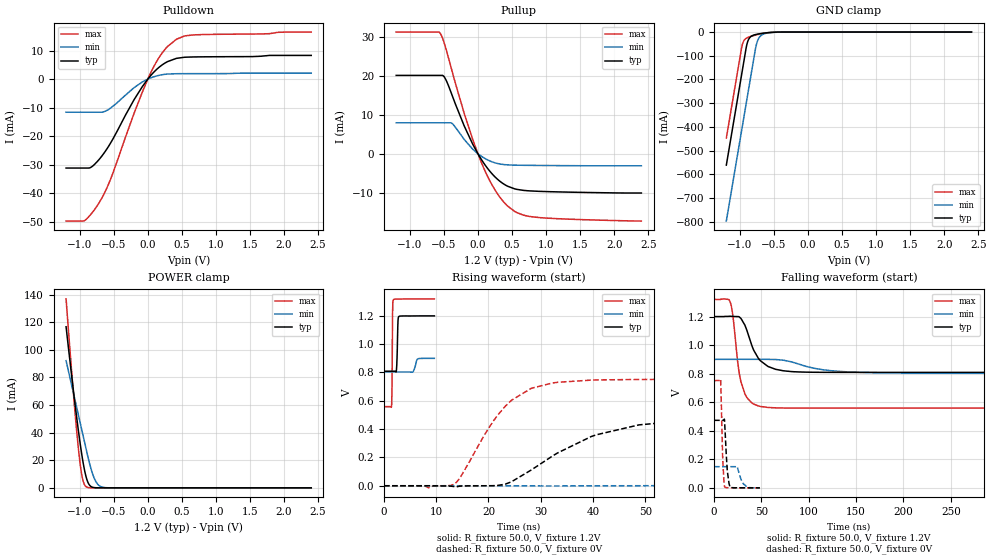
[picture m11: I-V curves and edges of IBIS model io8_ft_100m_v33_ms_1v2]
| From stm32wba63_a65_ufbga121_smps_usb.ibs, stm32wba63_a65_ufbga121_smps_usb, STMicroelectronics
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[Model]   io8_ft_100m_v33_ms_1v2
Model_type I/O
Polarity   Non-Inverting
Enable   Active-Low
| CAP_THRESHOLD on pad IOFT is "UDTCAPC" :
| Rising=30.0% of vddiom   Falling=70.0% of vddiom
| C_comp min and max val. don't necessarily correlate with the min and max pvt
| but are the smallest and greatest pad capacitance found.
| var   typ   min   max
C_comp   2.93788pF  2.85554pF  3.04885pF
|C_comp_pullup   1.70472pF  1.54555pF  1.84622pF
|C_comp_pulldown   1.23316pF  1.30998pF  1.20263pF
Vinl = 450.0mV
Vinh = 660.0mV
Vmeas = 600.0mV   | Reference voltage for timing measurements
Cref  = 50.0pF   | Timing specification test load capacitance value
Rref  = 1.0MOhm   | Timing specification test load resistance value
Vref  = 660.0mV   | Timing specification test load voltage
[Model Spec]
| TIME_THRESHOLD on pin ZIV33M is "CMOS" :
| Rising=50.0% of vddiom   Falling=50.0% of vddiom
Vinl 436.50000mV 331.50000mV 482.50000mV
Vinh 753.50000mV 549.50000mV 837.50000mV
| variable   typ   min   max
[Temperature Range] 25.0 140.0 -40.0
| variable   typ   min   max
[Voltage Range] 1.2V 900.0mV 1.32V
| variable   typ   min   max
[POWER Clamp Reference] 1.2V 900.0mV 1.32V
| variable   typ   min   max
[GND Clamp Reference] 0V 0V 0V
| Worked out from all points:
|   slope of the pulldown table from 0 to 0.18 V, typ, clamps not added: 40.6 ohm
|   slope of the pullup table from 0 to 0.18 V, typ, clamps not added: 39.4 ohm
|   GND clamp passes 1 mA (typ) near -0.51 V on its own axis
|   POWER clamp passes 1 mA (typ) near -0.83 V on its own axis
|   rising waveform, R_fixture 50.0, V_fixture 1.2V: 20-80 % time 157ps typ, 430ps min, 91ps max; typ from 0.809 V to 1.2 V
|   falling waveform, R_fixture 50.0, V_fixture 1.2V: 20-80 % time 16ns typ, 38ns min, 9.4ns max; typ from 1.2 V to 0.809 V
|   rising waveform, R_fixture 50.0, V_fixture 0V: 20-80 % time 15.4ns typ, 36.4ns min, 8.28ns max; typ from 0 V to 0.473 V
|   falling waveform, R_fixture 50.0, V_fixture 0V: 20-80 % time 2.69ns typ, 5.04ns min, 1.95ns max; typ from 0.473 V to 0 V
[POWER Clamp]
-1.2V     116.7mA    92.13mA    136.9mA
-1.09V    69.42mA    68.21mA    67.14mA
-1.02V    41.75mA    52.99mA    28.91mA
-990mV    30.98mA    46.47mA    16.09mA
-970mV    24.36mA    42.12mA    9.575mA
-940mV    15.59mA    35.6mA     3.485mA
-910mV    8.693mA    29.07mA    1.01mA
-860mV    2.259mA    18.59mA    104.6uA
-780mV    143.1uA    6.246mA    2.555uA
-720mV    16.22uA    1.846mA    157.1nA
-650mV    1.267uA    330.3uA    6.118nA
2.4V      0A         0A         0A
[GND Clamp]
-1.2V     -561.6mA   -797.4mA   -447.4mA
-980mV    -187.6mA   -423.4mA   -73.43mA
-960mV    -153.6mA   -389.4mA   -48.26mA
-900mV    -54.17mA   -287.4mA   -24.97mA
-870mV    -29.55mA   -236.4mA   -21.19mA
-830mV    -17.05mA   -168.4mA   -17.42mA
-760mV    -9.921mA   -54.55mA   -11.89mA
-730mV    -8.191mA   -29.78mA   -9.811mA
-690mV    -6.26mA    -14.49mA   -7.318mA
-600mV    -2.976mA   -4.315mA   -3.058mA
-380mV    -57.63uA   -251uA     -19.49uA
2.4V      872.7pA    204.8nA    349.4pA
| variable   typ   min   max
[Pullup Reference] 1.2V 900.0mV 1.32V
| variable   typ   min   max
[Pulldown Reference] 0V 0V 0V
[Pullup]
-1.2V     20.06mA    7.937mA    31.16mA
-580mV    20.06mA    7.937mA    31.16mA
-550mV    20.06mA    7.937mA    30.73mA
-480mV    19.26mA    7.937mA    27.49mA
-380mV    15.01mA    7.757mA    21.16mA
-200mV    7.069mA    3.64mA     10.26mA
20mV      -590.5uA   -260.8uA   -901.4uA
230mV     -5.55mA    -2.199mA   -8.66mA
440mV     -8.335mA   -2.843mA   -13.44mA
570mV     -9.105mA   -2.921mA   -15.05mA
790mV     -9.528mA   -2.972mA   -16.12mA
2.4V      -10.04mA   -3.075mA   -17.21mA
[Pulldown]
-1.2V     -31.2mA    -11.62mA   -49.78mA
-930mV    -31.2mA    -11.62mA   -49.64mA
-830mV    -30.86mA   -11.62mA   -47.25mA
-710mV    -28.04mA   -11.62mA   -43.19mA
-550mV    -22.55mA   -10.2mA    -35.3mA
-200mV    -7.146mA   -2.964mA   -11.89mA
40mV      1.171mA    405.8uA    2.092mA
130mV     3.416mA    1.118mA    6.182mA
230mV     5.302mA    1.613mA    9.763mA
420mV     7.288mA    1.898mA    13.99mA
670mV     7.779mA    1.924mA    15.51mA
2.4V      8.319mA    2.103mA    16.52mA
[Ramp]
dV/dt_r 283.79316mV/14.69967ns 88.92959mV/36.11555ns 450.99229mV/8.2606ns
dV/dt_f 234.65981mV/15.76017ns 57.89579mV/37.90378ns 456.73588mV/9.06629ns
R_load = 50.0
| Removed startup time: 0s 0s 0s  .
| Removed end time: 9.65ns.
[Rising Waveform]
R_fixture   = 50.0
V_fixture   = 1.2V
V_fixture_min = 900.0mV
V_fixture_max = 1.32V
0s        808.9mV    803.5mV    558.8mV
1.45ns    808.9mV    803.5mV    557mV
1.55ns    808.9mV    803.5mV    716.3mV
1.65ns    808.9mV    803.5mV    1.222V
1.8ns     808.9mV    803.5mV    1.313V
2.4ns     820.8mV    803.5mV    1.318V
2.5ns     896.9mV    803.5mV    1.319V
2.65ns    1.127V     803.5mV    1.319V
2.8ns     1.193V     803.5mV    1.318V
9.65ns    1.2V       899.8mV    1.32V
| Removed startup time: 0s 0s 0s  .
| Removed end time: 398.4ns.
[Falling Waveform]
R_fixture   = 50.0
V_fixture   = 1.2V
V_fixture_min = 900.0mV
V_fixture_max = 1.32V
0s        1.2V       900mV      1.32V
17.05ns   1.202V     900mV      1.301V
19.6ns    1.201V     900mV      1.218V
25.3ns    1.2V       900.6mV    863.7mV
28.4ns    1.187V     900.6mV    741.7mV
34.65ns   1.103V     900.5mV    632.4mV
46.8ns    907.1mV    900.2mV    573.8mV
84.95ns   813.2mV    876.4mV    558.9mV
146.4ns   808.9mV    811.1mV    558.8mV
398.4ns   808.9mV    803.5mV    558.8mV
| Removed startup time: 0s 0s 0s  .
| Removed end time: 398.35ns.
[Rising Waveform]
R_fixture   = 50.0
V_fixture   = 0V
V_fixture_min = 0V
V_fixture_max = 0V
0s        4.831nV    215.5nV    3.391nV
13.25ns   -4.891mV   183nV      8.354mV
20.8ns    235uV      21.56nV    449.3mV
24.4ns    27.96mV    22.17uV    603.6mV
28.2ns    111.6mV    -705.9uV   688.3mV
39.65ns   347.3mV    -123.2uV   746.2mV
48.8ns    429.9mV    96.97uV    750.7mV
73.2ns    470.6mV    30.18mV    751.6mV
138.2ns   472.9mV    141.2mV    751.6mV
398.4ns   473mV      148.2mV    751.7mV
| Removed startup time: 0s 0s 0s  .
| Removed end time: 48.4ns.
[Falling Waveform]
R_fixture   = 50.0
V_fixture   = 0V
V_fixture_min = 0V
V_fixture_max = 0V
0s        473mV      148.3mV    751.7mV
6.9ns     473mV      148.3mV    756.4mV
9.1ns     473mV      148.3mV    211.9mV
11.15ns   460.6mV    148.3mV    7.26mV
13.85ns   130.1mV    148.3mV    1.37mV
16.8ns    5.538mV    148.3mV    823.3uV
23.95ns   492.3uV    151.9mV    280.4uV
29.65ns   445.5uV    40.98mV    127.3uV
34.6ns    281.7uV    8.485mV    68.62uV
48.4ns    91.04uV    259.4uV    11.72uV
